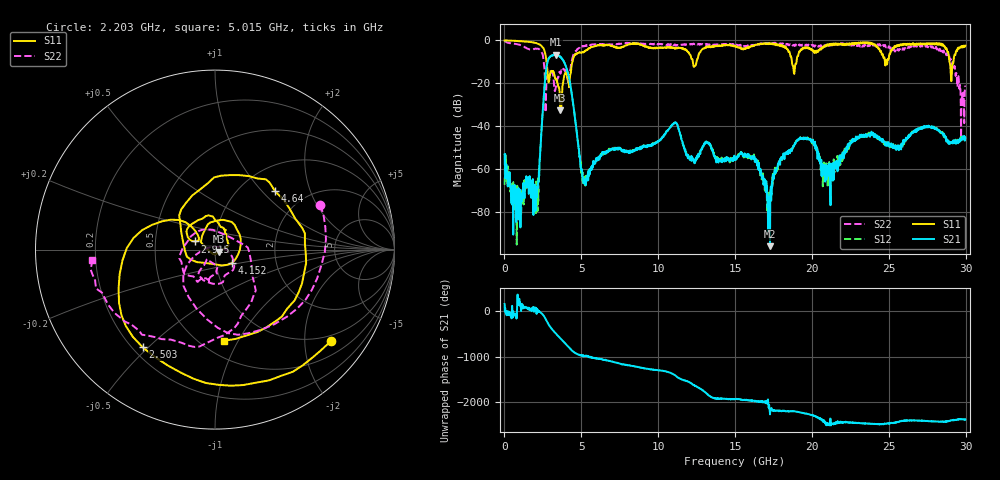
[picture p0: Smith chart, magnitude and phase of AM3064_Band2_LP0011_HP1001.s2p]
# Hz S DB R 50.0
!freq dBS11 angS11 dBS21 angS21 dBS12 angS12 dBS22 angS22
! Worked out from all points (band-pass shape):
!   1600 points, 10 MHz to 29.98 GHz, reference 50 ohm
!   highest |S21| = -6.62 dB at 3.328 GHz (marker M1); lowest = -95.8 dB at 17.27 GHz (marker M2)
!   |S21| within 3 dB of the highest: 2.818 GHz to 3.844 GHz (1.027 GHz wide, 30.8 % of centre)
!   lowest |S11| = -32.6 dB at 3.628 GHz (marker M3), VSWR 1.05, Z = 52.1 - j1.18 ohm
!   |S11| at or under -10 dB: 2.737 GHz to 4.424 GHz (1.687 GHz wide, 47.1 % of centre); 18.7 GHz to 19 GHz (298 MHz wide, 1.58 % of centre); 28.95 GHz to 29.2 GHz (255.6 MHz wide, 0.879 % of centre)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
!   |S22| runs from -45.4 to -0.2 dB; largest |S21 - S12| = 0.016
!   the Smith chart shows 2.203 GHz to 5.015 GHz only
!   S11 on the Smith chart (normalised r, x): 2.203 GHz: 0.85, -2.67; 2.503 GHz: 0.24, -0.48; 2.915 GHz: 0.79, +0.07; 4.152 GHz: 1.19, -0.18; 4.64 GHz: 1.42, +1.19; 5.015 GHz: 0.64, -0.88
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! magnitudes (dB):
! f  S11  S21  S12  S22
! 10 MHz  -0.1  -53.1  -67.2  -0.2
! 909.7 MHz  -0.4  -68.7  -73.2  -2.0
! 2.203 GHz  -1.7  -65.6  -74.8  -3.9
! 2.503 GHz  -3.4  -31.6  -31.5  -7.2
! 2.915 GHz  -18.3  -8.1  -8.0  -15.2
! 3.328 GHz  -17.8  -6.6  -6.7  -22.6
! 3.628 GHz  -32.6  -7.7  -7.5  -15.2
! 4.152 GHz  -18.4  -16.1  -16.0  -19.9
! 4.64 GHz  -6.6  -39.2  -39.0  -5.2
! 5.015 GHz  -5.8  -60.6  -59.6  -3.3
! 10 GHz  -3.5  -47.1  -46.9  -1.8
! 11.11 GHz  -4.0  -38.4  -38.3  -2.3
! 12.12 GHz  -7.2  -55.3  -54.6  -1.7
! 15 GHz  -2.7  -55.5  -55.3  -1.9
! 17.27 GHz  -1.5  -95.8  -71.0  -1.2
! 18.1 GHz  -2.7  -54.8  -54.7  -1.4
! 19.99 GHz  -4.3  -46.7  -47.0  -2.2
! 21.28 GHz  -1.7  -62.3  -63.7  -1.6
! 23.14 GHz  -1.1  -44.7  -44.7  -2.9
! 25 GHz  -8.5  -47.7  -48.7  -2.8
! 28.56 GHz  -2.5  -44.2  -44.6  -4.7
! 29.98 GHz  -2.4  -45.6  -46.5  -21.6
